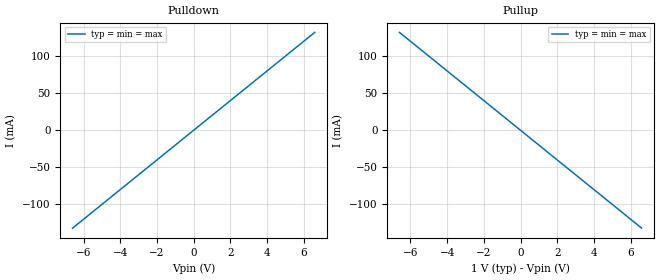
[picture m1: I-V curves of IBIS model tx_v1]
[IBIS Ver]   5.1
[File Name]   tusb564_v1.ibs
[File Rev]   1.0
[Component]   tusb564_v1
[Manufacturer] My Company
[Package]
R_pkg  0.0   NA   NA
L_pkg  0.0   NA   NA
C_pkg  0.0   NA   NA
[Pin]   signal_name   model_name   R_pin L_pin  C_pin
1p   tx_v1_p   tx_v1
1n   tx_v1_n   tx_v1
2p   tusb564_rx1_2p   tusb564_rx1
2n   tusb564_rx1_2n   tusb564_rx1
[Diff_Pin] inv_pin vdiff tdelay_typ tdelay_min tdelay_max
1p   1n   NA   NA   NA   NA
2p   2n   NA   NA   NA   NA
[Model] tusb564_rx1
Model_type Input
C_comp 0p 0p 0p
Vinh = 0.25
Vinl = -0.25
[Temperature_Range] 25 125 0
[Voltage Range] 1.0 1.0 1.0
[Algorithmic Model]
Executable Windows_cl18.00.40629_64 tusb564_rx1_x64.dll tusb564_rx1.ami
[End Algorithmic Model]
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| Models and submodels in the file (2): tx_v1 (Output), tusb564_rx1 (Input)
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[Model] tx_v1
Model_type Output
C_comp 0p 0p 0p
Cref = 0
Vref = 0.5
Rref = 50
Vmeas = 0.5
[Temperature_Range] 25 125 0
[Voltage Range] 1.0 1.0 1.0
[Algorithmic Model]
Executable Windows_cl18.00.40629_64 tx_v1_x64.dll tx_v1.ami
[End Algorithmic Model]
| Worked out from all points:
|   slope of the pulldown table from 0 to 0.15 V, typ, clamps not added: 50 ohm
|   slope of the pullup table from 0 to 0.15 V, typ, clamps not added: 50 ohm
[Pulldown]
-6.6V     -132mA     -132mA     -132mA
0V        0A         0A         0A
6.6V      132mA      132mA      132mA
[Pullup]
-6.6V     132mA      132mA      132mA
0V        0A         0A         0A
6.6V      -132mA     -132mA     -132mA
[GND Clamp]
-6.6V     0A         0A         0A
0V        0A         0A         0A
6.6V      0A         0A         0A
[Power Clamp]
-6.6V     0A         0A         0A
0V        0A         0A         0A
6.6V      0A         0A         0A
[Ramp]
dV/dt_r 0.3/1.5p 0.3/1.5p 0.3/1.5p
dV/dt_f 0.3/1.5p 0.3/1.5p 0.3/1.5p
